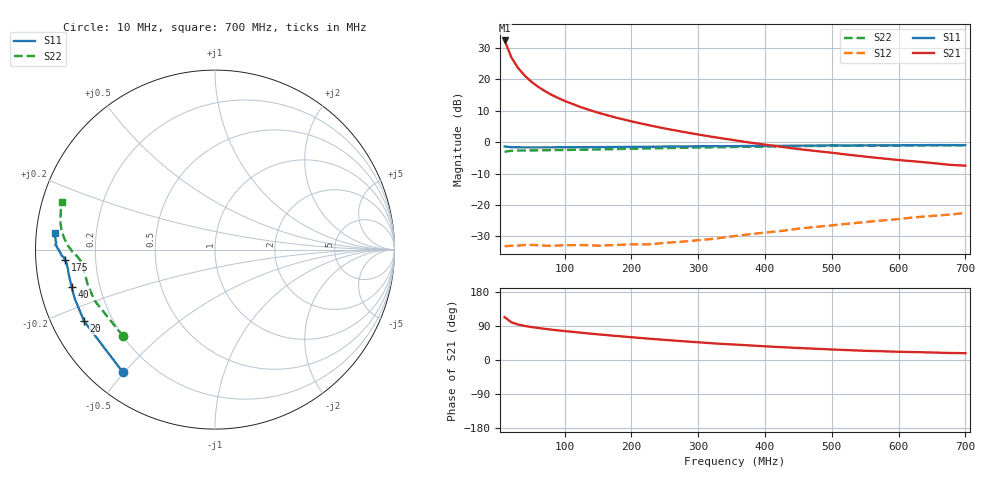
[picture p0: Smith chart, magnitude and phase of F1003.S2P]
! Date: Mon Aug 07 13:27:31 1995
# MHZ  S  MA  R  50.0000
!  POLYFET RF DEVICES
!  F1003
!  S PARAMETERS
!  VDS=28V, IDQ=600mA
!FREQ  S11MAG S11ANG S21MAG S21ANG S12MAG S12ANG S22MAG S22ANG
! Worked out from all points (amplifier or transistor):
!   34 points, 10 MHz to 700 MHz, reference 50 ohm
!   highest |S21| = 32.4 dB at 10 MHz (marker M1)
!   |S21| within 3 dB of that: start of sweep to 15.62 MHz
!   unconditionally stable (mu >= 1): 174.9 MHz to 482.3 MHz
!   at 60 MHz: K = 0.37, MSG = 25.3 dB, |S12| = -32.8 dB
!   at 300 MHz: K = 1.24, MAG = 13.9 dB, |S12| = -31.3 dB
!   at 700 MHz: K = 0.83, MSG = 7.5 dB, |S12| = -22.6 dB
!   S11 on the Smith chart (normalised r, x): 10 MHz: 0.10, -0.50; 20 MHz: 0.10, -0.25; 40 MHz: 0.10, -0.13; 175 MHz: 0.09, -0.03; 700 MHz: 0.05, +0.05
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10  0.8549 -126.9  41.78 113.1  0.02201 27.5  0.7038 -136.5
20  0.8312 -151.3  22.61 99.6  0.0223 16.4  0.7289 -157.1
30  0.828 -160.6  15.28 93.8  0.02246 12.4  0.7353 -164.5
40  0.8257 -165.3  11.5 89.9  0.02299 10.8  0.7366 -168.2
50  0.8251 -168.1  9.202 87.0  0.02303 10.7  0.74 -170.6
60  0.826 -170.0  7.656 84.5  0.02282 11.4  0.741 -172.1
70  0.8268 -171.3  6.547 82.3  0.02245 12.2  0.743 -173.4
80  0.8263 -172.5  5.703 80.1  0.02231 12.4  0.7454 -174.0
90  0.8285 -173.2  5.064 78.2  0.02254 12.2  0.7484 -174.6
100  0.8277 -173.7  4.539 76.4  0.0228 14.8  0.7501 -175.1
125  0.8305 -174.8  3.586 71.9  0.02294 17.3  0.7585 -176.1
150  0.8346 -175.5  2.949 67.6  0.02245 21.7  0.7666 -177.0
175  0.8379 -176.1  2.488 63.8  0.02292 26.3  0.7753 -177.6
200  0.8418 -176.7  2.144 60.1  0.02353 31.1  0.7852 -178.5
225  0.8445 -177.3  1.873 56.4  0.02347 34.8  0.7943 -179.1
250  0.8519 -177.6  1.652 53.0  0.02482 39.6  0.8024 180.0
300  0.8591 -178.5  1.324 46.8  0.02737 47.5  0.8232 178.2
325  0.8614 -178.7  1.198 43.6  0.02898 51.0  0.8284 177.3
375  0.8693 -179.5  0.9927 38.7  0.03395 57.6  0.8437 175.5
475  0.8817 178.7  0.7243 29.8  0.04457 61.7  0.8669 171.5
600  0.89 176.0  0.5187 21.7  0.05955 63.1  0.8842 166.5
700  0.897 174.2  0.4215 17.9  0.07435 61.7  0.8929 162.6
